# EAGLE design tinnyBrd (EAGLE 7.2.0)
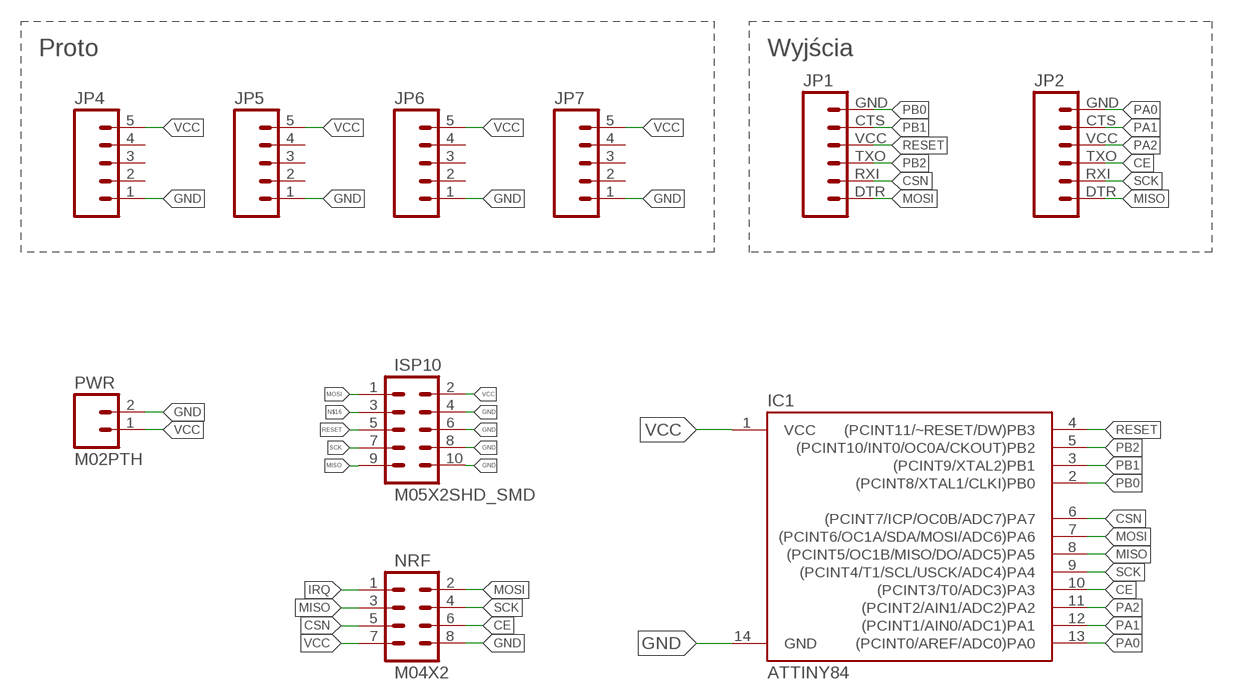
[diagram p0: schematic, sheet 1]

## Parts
IC1  ATTINY84  [SO14]
ISP10  M05X2SHD_SMD  [2X5-SHROUDED_SMD]
JP1  M06SIP  [1X06]
JP2  M06SIP  [1X06]
JP4  M05PTH  [1X05]
JP5  M05PTH  [1X05]
JP6  M05PTH  [1X05]
JP7  M05PTH  [1X05]
NRF  M04X2  [2X4_SMD]
PWR  M02PTH  [1X02]

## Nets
CE: IC1.10((PCINT3/T0/ADC3)PA3) JP2.TXO NRF.6
CSN: IC1.6((PCINT7/ICP/OC0B/ADC7)PA7) JP1.RXI NRF.5
GND: IC1.14(GND) ISP10.4 ISP10.6 ISP10.8 ISP10.10 JP4.1 JP5.1 JP6.1 JP7.1 NRF.8 PWR.2
IRQ: NRF.1
MISO: IC1.8((PCINT5/OC1B/MISO/DO/ADC5)PA5) ISP10.9 JP2.DTR NRF.3
MOSI: IC1.7((PCINT6/OC1A/SDA/MOSI/ADC6)PA6) ISP10.1 JP1.DTR NRF.2
N$16: ISP10.3
PA0: IC1.13((PCINT0/AREF/ADC0)PA0) JP2.GND
PA1: IC1.12((PCINT1/AIN0/ADC1)PA1) JP2.CTS
PA2: IC1.11((PCINT2/AIN1/ADC2)PA2) JP2.VCC
PB0: IC1.2((PCINT8/XTAL1/CLKI)PB0) JP1.GND
PB1: IC1.3((PCINT9/XTAL2)PB1) JP1.CTS
PB2: IC1.5((PCINT10/INT0/OC0A/CKOUT)PB2) JP1.TXO
RESET: IC1.4((PCINT11/~RESET/DW)PB3) ISP10.5 JP1.VCC
SCK: IC1.9((PCINT4/T1/SCL/USCK/ADC4)PA4) ISP10.7 JP2.RXI NRF.4
VCC: IC1.1(VCC) ISP10.2 JP4.5 JP5.5 JP6.5 JP7.5 NRF.7 PWR.1
Unconnected: JP4.2 JP4.3 JP4.4 JP5.2 JP5.3 JP5.4 JP6.2 JP6.3 JP6.4 JP7.2 JP7.3 JP7.4

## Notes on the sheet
- Proto | Wyjścia

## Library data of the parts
IC1 = SparkFun-DigitalIC:ATTINY84: Atmel 14-pin 2/4/8kB flash uC; PROD_ID: IC-11285
ISP10 = SparkFun-Connectors:M05X2: Header 5x2 Standard 10-pin dual row 0.1" header. Commonly used with AVR-ISP. Use with Spark Fun Electronics SKU: PRT-00778
JP1 JP2 = SparkFun-Connectors:M06: Header 6 Standard 6-pin 0.1" header. Use with straight break away headers (SKU : PRT-00116), right angle break away headers (PRT-00553), swiss pins (PRT-00743), machine pins (PRT-00117), and female headers (PRT-00115). Molex polarized connector foot print use with SKU : PRT-08094 with associated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
JP4-JP7 = SparkFun-Connectors:M05: Header 5 Standard 5-pin 0.1" header. Use with straight break away headers (SKU : PRT-00116), right angle break away headers (PRT-00553), swiss pins (PRT-00743), machine pins (PRT-00117), and female headers (PRT-00115). Molex polarized connector foot print use with SKU : PRT-08230 with associated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
NRF = nettigo:M04X2
PWR = SparkFun-Connectors:M02: Standard 2-pin 0.1" header. Use with

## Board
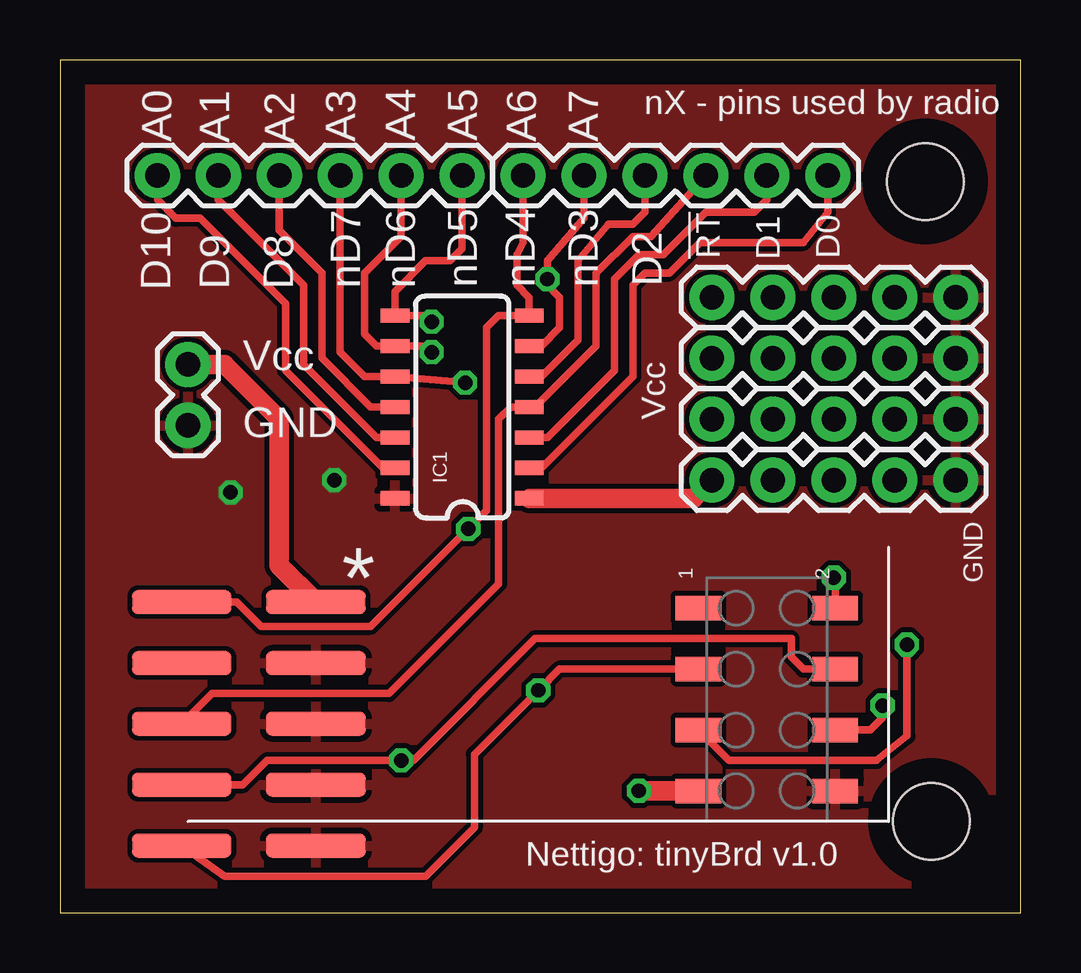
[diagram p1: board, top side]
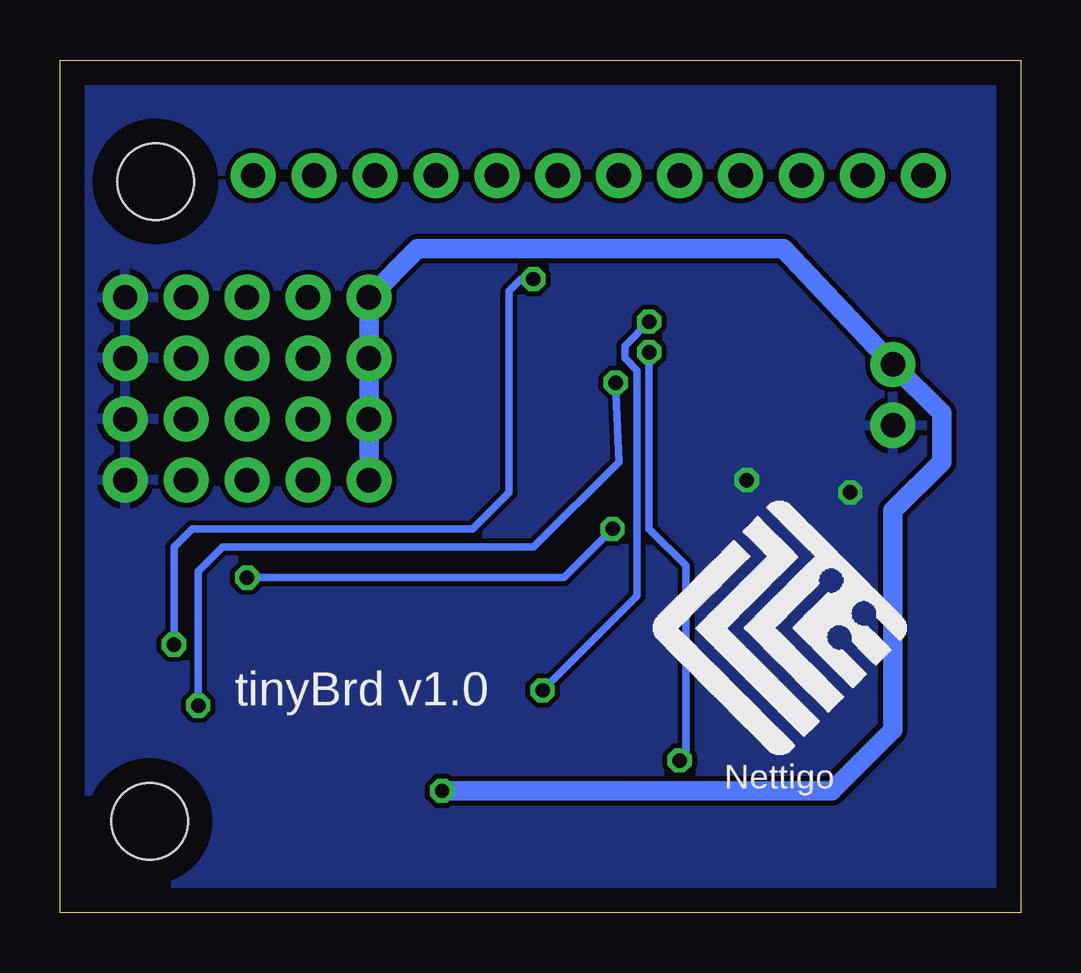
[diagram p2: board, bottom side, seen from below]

Size 40.06 x 35.55 mm. Coordinates in mm from the lower left corner, seen from the top.
Outline: 0,0 40.06,0 40.06,35.55 0,35.55 0,0
Copper layers (1*16): Top 0.035mm / dielectric 1.5mm / Bottom 0.035mm
Design rules "default": minimum track width 10mil, minimum drill 24mil, track to track 8mil, track to pad 8mil, pad to pad 8mil, via to via 8mil, smd to smd 8mil, copper to edge 40mil, drill to drill 8mil, minimum pad ring 10mil, minimum via ring 8mil, stop-mask expansion 4mil, vias tented up to drill 0mil, thermal gap 10mil
Holes 3.2 mm at 36.32,3.81 36.07,30.48

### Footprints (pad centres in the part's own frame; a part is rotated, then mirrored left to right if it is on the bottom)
SO14 = smd 0.6 x 1.2: 1 -3.81,-2.8; 2 -2.54,-2.8; 3 -1.27,-2.8; 4 0,-2.8; 5 1.27,-2.8; 6 2.54,-2.8; 7 3.81,-2.8; 8 3.81,2.8; 9 2.54,2.8; 10 1.27,2.8; 11 0,2.8; 12 -1.27,2.8; 13 -2.54,2.8; 14 -3.81,2.8
2X5-SHROUDED_SMD = smd 4.15 x 1: 1 -2.794,5.08; 2 2.794,5.08; 3 -2.794,2.54; 4 2.794,2.54; 5 -2.794,0; 6 2.794,0; 7 -2.794,-2.54; 8 2.794,-2.54; 9 -2.794,-5.08; 10 2.794,-5.08
1X06 = drill 1.016 pad 1.88: CTS 10.16,0; DTR 0,0; GND 12.7,0; RXI 2.54,0; TXO 5.08,0; VCC 7.62,0
1X05 = drill 1.016 pad 1.88: 1 0,0; 2 2.54,0; 3 5.08,0; 4 7.62,0; 5 10.16,0
2X4_SMD = smd 1.02 x 1.9: 1 -3.81,-2.85; 2 -3.81,2.85; 3 -1.27,-2.85; 4 -1.27,2.85; 5 1.27,-2.85; 6 1.27,2.85; 7 3.81,-2.85; 8 3.81,2.85
1X02 = drill 1.016 pad 1.88: 1 0,0; 2 2.54,0

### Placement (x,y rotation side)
IC1  16.76,21.08 90 top
ISP10  7.87,7.87 0 top
JP1  19.3,30.73 0 top
JP2  16.76,30.73 180 top
JP4  37.34,25.65 180 top
JP5  37.34,23.11 180 top
JP6  37.34,20.57 180 top
JP7  37.34,18.03 180 top
NRF  29.46,8.89 270 top
PWR  5.33,22.86 270 top

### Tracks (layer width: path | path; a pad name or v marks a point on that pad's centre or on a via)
CE  (via drill 0.6)
  Top 0.305: JP2.TXO 11.68,23.37 12.7,22.35 IC1.10 v16.89,22.1 | v34.29,8.64 34.29,8.13 33.78,7.62 NRF.6
  Bottom 0.305: v16.89,22.1 16.76,18.8 20.32,15.24 33.27,15.24 34.29,14.22 v34.29,8.64
CSN  (via drill 0.6)
  Top 0.305: IC1.6 20.07,23.62 20.83,24.38 20.83,25.65 20.32,26.16 v20.32,26.42 20.32,27.18 21.84,28.96 JP1.RXI | NRF.5 27.88,6.35 34.04,6.35 35.31,7.37 v35.31,11.18
  Bottom 0.305: v35.31,11.18 35.31,15.24 34.54,16 22.86,16 21.34,17.53 21.34,25.91 20.83,26.42 v20.32,26.42
GND  (via drill 0.6)
  other vias: 11.43,18.03 7.11,17.53
  pour Top: -0.25,35.9 40.39,35.81 40.39,-0.51 0,0
  pour Bottom: 0.55,35.65 0,-0.51 40.39,-0.51 40.39,35.18
MISO  (via drill 0.6)
  Top 0.305: JP2.DTR 16.76,27.69 16.26,27.18 15.24,27.18 13.96,25.9 IC1.8 15.24,24.89 v15.49,24.64 | NRF.3 20.83,10.16 v19.94,9.27 17.27,6.6 17.27,3.56 15.24,1.52 6.86,1.52 ISP10.9
  Bottom 0.305: v15.49,24.64 16.51,23.62 16.51,23.11 16,22.61 16,13.21 v19.94,9.27
MOSI  (via drill 0.6)
  Top 0.305: ISP10.1 7.37,12.95 8.38,11.94 12.95,11.94 v17.02,16 17.78,16.76 17.78,24.38 18.29,24.89 IC1.7 19.56,25.65 19.05,26.16 19.05,27.43 19.3,27.94 JP1.DTR | NRF.2 32.31,13.91 v32.26,13.97
  Bottom 0.305: v32.26,13.97 19.05,13.97 v17.02,16
PA0
  Top 0.305: IC1.13 13.46,18.54 9.4,22.61 9.4,25.4 5.84,28.96 4.83,28.96 4.06,29.72 JP2.GND
PA1
  Top 0.305: IC1.12 13.21,19.81 10.16,22.86 10.16,26.16 6.6,29.72 JP2.CTS
PA2
  Top 0.305: IC1.11 12.95,21.08 10.92,23.11 10.92,26.67 9.14,28.45 JP2.VCC
PB0
  Top 0.305: IC1.2 20.07,18.54 23.88,22.35 23.88,26.16 24.38,26.67 25.4,26.67 26.67,27.94 30.99,27.94 32,29.21 JP1.GND
PB1
  Top 0.305: IC1.3 20.32,19.81 23.11,22.61 23.11,26.42 24.13,27.43 25.15,27.43 26.92,29.21 28.96,29.21 29.46,29.72 JP1.CTS
PB2
  Top 0.305: IC1.5 20.07,22.35 21.59,23.88 21.59,27.18 22.86,28.7 23.88,28.7 24.38,29.21 JP1.TXO
RESET
  Top 0.305: ISP10.5 6.35,9.14 13.72,9.14 18.29,13.72 18.29,20.57 18.8,21.08 IC1.4 19.81,21.08 22.35,23.62 22.35,26.67 23.88,28.19 24.64,28.19 JP1.VCC
SCK  (via drill 0.6)
  Top 0.305: JP2.RXI 14.22,28.19 12.7,26.67 12.7,24.13 13.21,23.62 IC1.9 15.24,23.62 v15.49,23.37 | NRF.4 30.99,10.16 30.48,10.67 30.48,11.43 19.81,11.43 14.73,6.35 v14.22,6.35 8.64,6.35 7.62,5.33 ISP10.7
  Bottom 0.305: v15.49,23.37 15.49,16 13.97,14.48 13.97,6.6 v14.22,6.35
VCC  (via drill 0.6)
  Top 0.813: JP7.5 26.42,17.27 IC1.1 | ISP10.2 9.14,14.48 9.14,20.57 6.86,22.86 PWR.1 | NRF.7 v24.13,5.08
  Bottom 0.813: JP7.5 JP6.5 JP5.5 JP4.5 25.15,27.69 9.91,27.69 PWR.1 3.3,20.83 3.3,18.8 5.33,16.76 5.33,7.62 7.87,5.08 v24.13,5.08

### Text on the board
tNames: nX - pins used by radio | A0 | A1 | A2 | A3 | A4 | A5 | A6 | A7 | !RT | D1 | D0 | D10 | D9 | D8 | nD7 | nD6 | nD5 | nD4 | nD3 | D2 | Vcc | Vcc | GND | GND | * | Nettigo: tinyBrd v1.0
bNames: tinyBrd v1.0 | Nettigo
